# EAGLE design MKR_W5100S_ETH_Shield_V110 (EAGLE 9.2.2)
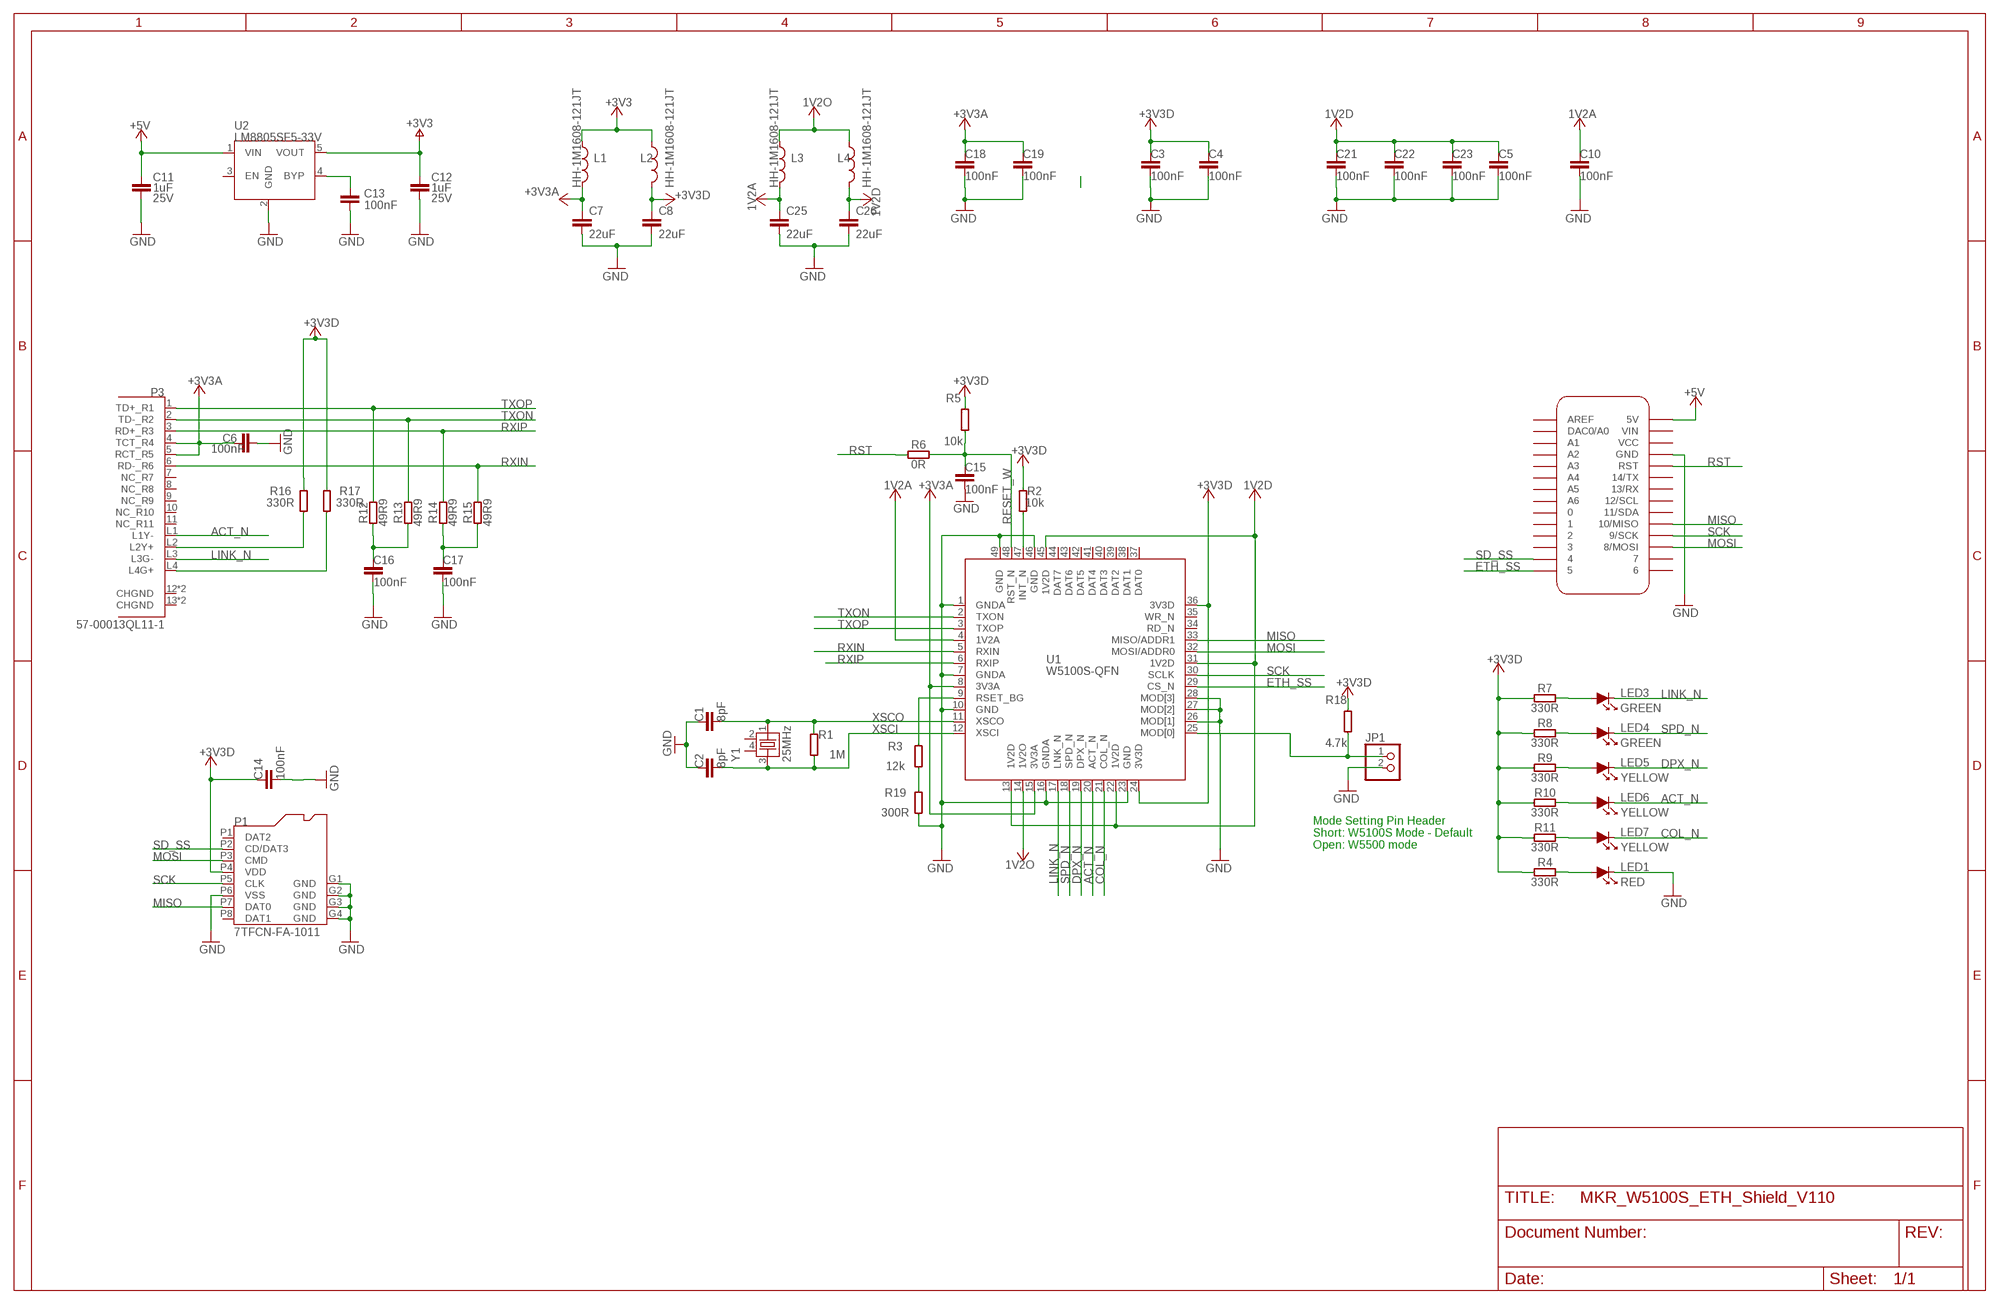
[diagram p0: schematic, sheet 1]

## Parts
C1  8pF  C-1UF-0402  [0402-1005X55N]
C2  8pF  C-1UF-0402  [0402-1005X55N]
C3  100nF  C-1UF-0402  [0402-1005X55N]
C4  100nF  C-1UF-0402  [0402-1005X55N]
C5  100nF  C-1UF-0402  [0402-1005X55N]
C6  100nF  C-1UF-0402  [0402-1005X55N]
C7  22uF  C-22U-0805  [0805-R2013X50N]
C8  22uF  C-22U-0805  [0805-R2013X50N]
C10  100nF  C-1UF-0402  [0402-1005X55N]
C11  1uF  C-1UF-0402  [0402-1005X55N]
C12  1uF  C-1UF-0402  [0402-1005X55N]
C13  100nF  C-100NF-0402  [0402-1005X55N]
C14  100nF  C-1UF-0402  [0402-1005X55N]
C15  100nF  C-1UF-0402  [0402-1005X55N]
C16  100nF  C-1UF-0402  [0402-1005X55N]
C17  100nF  C-1UF-0402  [0402-1005X55N]
C18  100nF  C-1UF-0402  [0402-1005X55N]
C19  100nF  C-1UF-0402  [0402-1005X55N]
C21  100nF  C-1UF-0402  [0402-1005X55N]
C22  100nF  C-1UF-0402  [0402-1005X55N]
C23  100nF  C-1UF-0402  [0402-1005X55N]
C25  22uF  C-22U-0805  [0805-R2013X50N]
C26  22uF  C-22U-0805  [0805-R2013X50N]
JP1  PINHD-1X2  [1X02]
L1  HH-1M1608-121JT  BLM18PG471SN1D  [0603-1608X90N]
L2  HH-1M1608-121JT  BLM18PG471SN1D  [0603-1608X90N]
L3  HH-1M1608-121JT  BLM18PG471SN1D  [0603-1608X90N]
L4  HH-1M1608-121JT  BLM18PG471SN1D  [0603-1608X90N]
LED1  RED  LED-1608  [LED-1608]
LED3  GREEN  LED-1608  [LED-1608]
LED4  GREEN  LED-1608  [LED-1608]
LED5  YELLOW  LED-1608  [LED-1608]
LED6  YELLOW  LED-1608  [LED-1608]
LED7  YELLOW  LED-1608  [LED-1608]
MKR1  DNP  ARDUINO-UTILITY_MKRBOARDNO-OUTLINE  [ARDUINO-UTILITY_MKRBOARD-NOOUTLINE]
P1  7TFCN-FA-1011  [7TFCN-FA-1011]
P3  57-00013QL11-1  [57-00013QL11-1]
R1  1M  R-330R-0402  [0402-1005X55N]
R2  10k  R-330R-0402  [0402-1005X55N]
R3  12k  R-330R-0402  [0402-1005X55N]
R4  330R  R-330R-0402  [0402-1005X55N]
R5  10k  R-330R-0402  [0402-1005X55N]
R6  0R  R-330R-0402  [0402-1005X55N]
R7  330R  R-330R-0402  [0402-1005X55N]
R8  330R  R-330R-0402  [0402-1005X55N]
R9  330R  R-330R-0402  [0402-1005X55N]
R10  330R  R-330R-0402  [0402-1005X55N]
R11  330R  R-330R-0402  [0402-1005X55N]
R12  49R9  R-330R-0402  [0402-1005X55N]
R13  49R9  R-330R-0402  [0402-1005X55N]
R14  49R9  R-330R-0402  [0402-1005X55N]
R15  49R9  R-330R-0402  [0402-1005X55N]
R16  330R  R-330R-0402  [0402-1005X55N]
R17  330R  R-330R-0402  [0402-1005X55N]
R18  4.7k  R-330R-0402  [0402-1005X55N]
R19  300R  R-330R-0402  [0402-1005X55N]
U1  W5100S-QFN  [W5100S-QFN]
U2  LM8805SF5-33V  [SOT23-5L]
Y1  25MHz  XTAL3225  [XTAL3225]

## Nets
1V2A: C10.1 C25.1 L3.2 U1.4(1V2A)
1V2D: C5.1 C21.1 C22.1 C23.1 C26.1 L4.2 U1.13(1V2D) U1.22(1V2D) U1.31(1V2D) U1.45(1V2D)
1V2O: L3.1 L4.1 U1.14(1V2O)
+3V3 [power]: C12.1 L1.1 L2.1 U2.5(VOUT)
+3V3A [power]: C6.1 C7.1 C18.1 C19.1 L1.2 P3.4(TCT_R4) P3.5(RCT_R5) U1.8(3V3A) U1.15(3V3A)
+3V3D: C3.1 C4.1 C8.1 C14.1 L2.2 P1.P4(VDD) R2.1 R4.2 R5.2 R7.2 R8.2 R9.2 R10.2 R11.2 R16.1 R17.1 R18.2 U1.24(3V3D) U1.36(3V3D)
+5V: C11.1 MKR1.5V U2.1(VIN)
ACT_N: LED6.K P3.L1(L1Y-) U1.20(ACT_N)
COL_N: LED7.K U1.21(COL_N)
DPX_N: LED5.K U1.19(DPX_N)
ETH_SS: MKR1.5 U1.29(CS_N)
GND [gnd]: C1.1 C2.1 C3.2 C4.2 C5.2 C6.2 C7.2 C8.2 C10.2 C11.2 C12.2 C13.2 C14.2 C15.2 C16.2 C17.2 C18.2 C19.2 C21.2 C22.2 C23.2 C25.2 C26.2 JP1.2 LED1.K MKR1.GND P1.G1(GND) P1.G2(GND) P1.G3(GND) P1.G4(GND) P1.P6(VSS) R19.1 U1.1(GNDA) U1.7(GNDA) U1.10(GND) U1.16(GNDA) U1.23(GND) U1.26(MOD[1]) U1.27(MOD[2]) U1.28(MOD[3]) U1.46(GND) U1.49(GND) U2.2(GND)
LINK_N: LED3.K P3.L3(L3G-) U1.17(LNK_N)
MISO: MKR1.10(10/MISO) P1.P7(DAT0) U1.33(MISO/ADDR1)
MOSI: MKR1.8(8/MOSI) P1.P3(CMD) U1.32(MOSI/ADDR0)
N$1: LED3.A R7.1
N$2: P3.L2(L2Y+) R16.2
N$3: LED1.A R4.1
N$4: LED4.A R8.1
N$5: LED5.A R9.1
N$6: LED6.A R10.1
N$7: LED7.A R11.1
N$8: P3.L4(L4G+) R17.2
N$9: JP1.1 R18.1 U1.25(MOD[0])
N$11: C13.1 U2.4(BYP)
N$12: C16.1 R12.2 R13.2
N$13: R3.1 R19.2
N$15: C17.1 R14.2 R15.2
N$16: R2.2 U1.47(INT_N)
N$20: R3.2 U1.9(RSET_BG)
RESET_W: C15.1 R5.1 R6.1 U1.48(RST_N)
RST: MKR1.RST R6.2
RXIN: P3.6(RD-_R6) R15.1 U1.5(RXIN)
RXIP: P3.3(RD+_R3) R14.1 U1.6(RXIP)
SCK: MKR1.9(9/SCK) P1.P5(CLK) U1.30(SCLK)
SD_SS: MKR1.4 P1.P2(CD/DAT3)
SPD_N: LED4.K U1.18(SPD_N)
TXON: P3.2(TD-_R2) R13.1 U1.2(TXON)
TXOP: P3.1(TD+_R1) R12.1 U1.3(TXOP)
XSCI: C2.2 R1.1 U1.12(XSCI) Y1.3
XSCO: C1.2 R1.2 U1.11(XSCO) Y1.1
Unconnected: MKR1.0 MKR1.1 MKR1.2 MKR1.3 MKR1.6 MKR1.7 MKR1.11(11/SDA) MKR1.12(12/SCL) MKR1.13(13/RX) MKR1.14(14/TX) MKR1.A0(DAC0/A0) MKR1.A1 MKR1.A2 MKR1.A3 MKR1.A4 MKR1.A5 MKR1.A6 MKR1.AREF MKR1.VCC MKR1.VIN P1.P1(DAT2) P1.P8(DAT1) P3.7(NC_R7) P3.8(NC_R8) P3.9(NC_R9) P3.10(NC_R10) P3.11(NC_R11) P3.12(CHGND) P3.13(CHGND) P3.P$3(CHGND) P3.P$4(CHGND) U1.34(RD_N) U1.35(WR_N) U1.37(DAT0) U1.38(DAT1) U1.39(DAT2) U1.40(DAT3) U1.41(DAT4) U1.42(DAT5) U1.43(DAT6) U1.44(DAT7) U2.3(EN) Y1.2 Y1.4

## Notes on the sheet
- Mode Setting Pin Header
  Short: W5100S Mode - Default
  Open: W5500 mode

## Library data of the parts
C1-C6 C10-C12 C14-C19 C21-C23 = MK1_Zero:C: Capacitor; DESCR: CAP CER 1UF 25V 10% X5R 0402; MF: Murata; MPN: GRM155R61E105KA12D; VOLTAGE: 25V
C7 C8 C25 C26 = Arduino-rcl:C: SMD Capacitor; CODE-ARDUINO: 2233; DATASHEET: https://media.digikey.com/pdf/Data%20Sheets/Samsung%20PDFs/CL21A226MQCLQNC_character.pdf; DISTRIBUTOR-LINK: https://www.digikey.com/product-detail/en/samsung-electro-mechanics-america-inc/CL21A226MQCLQNC/1276-2412-1-ND/3890498; DISTRIBUTOR-PN: 1276-2412-1-ND; MANUFACTURER: Samsung; MANUFACTURER-PN: CL21A226MQCLQNC; VALUE: 22u
C13 = MK1_Zero:C: Capacitor; DESCR: CAP CER 0.1UF 50V 10% X5R 0402; MF: TDK; MPN: C1005X5R1H104K050BB
JP1 = PinHeader:PINHD-1X2: PIN HEADER
L1-L4 = MK1_Zero:BLM18PG471SN1D: FERRITE CHIP 470 OHM 1000MA 0603
LED1 LED3-LED7 = DIODE:LED-1608
MKR1 = MKRETHShieldV2.0:ARDUINO-UTILITY_MKRBOARD: MKR board footprint; DATASHEET: DNP; DISTRIBUTOR-LINK: DNP; DISTRIBUTOR-PN: DNP; MANUFACTURER: DNP; MANUFACTURER-PN: DNP
P1 = Connector:7TFCN-FA-1011
P3 = WIZnet:57-00013QL11-1
R1-R19 = MK1_Zero:R: Resistor; DESCR: RES 330 OHM 1/16W 1% 0402 SMD; MF: Yageo; MPN: RC0402FR-07330RL
U1 = WIZnet:W5100S-QFN
U2 = RECULATOR:LM8805SF5-33V
Y1 = X-TAL:XTAL3225

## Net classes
1 power: width 0.254 mm, drill 0.3 mm, clearance 0.127 mm
2 gnd: width 0.254 mm, drill 0.3 mm, clearance 0.127 mm

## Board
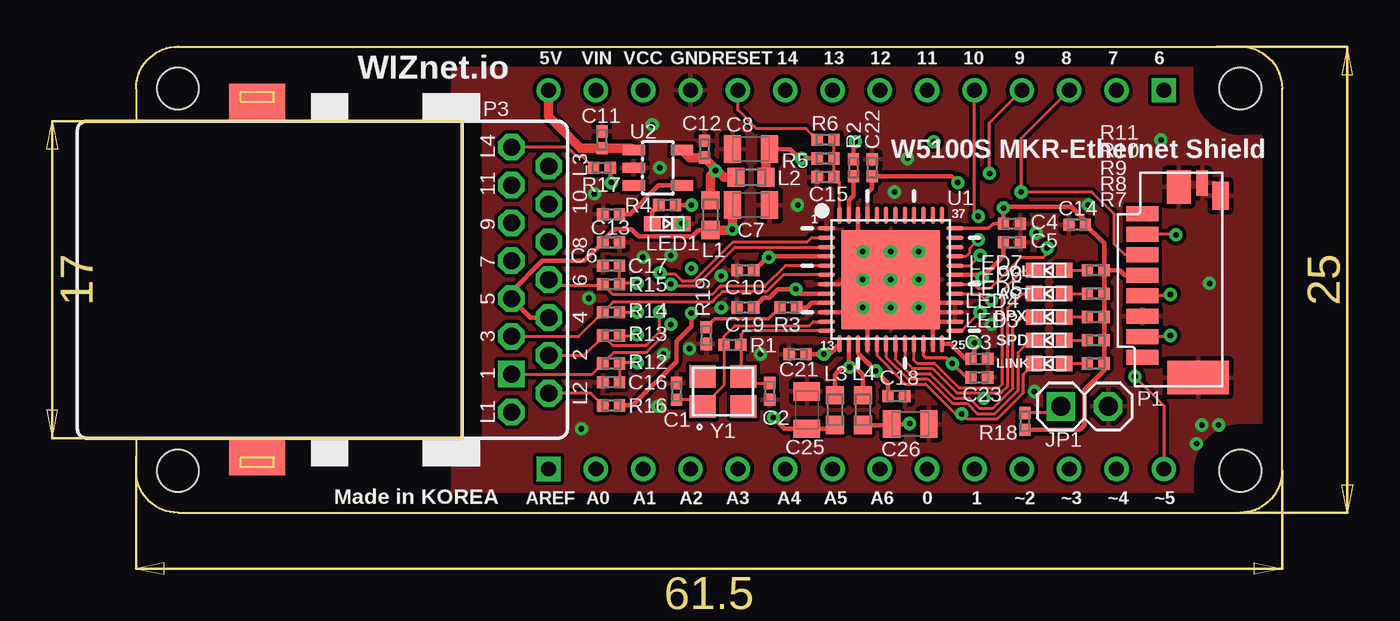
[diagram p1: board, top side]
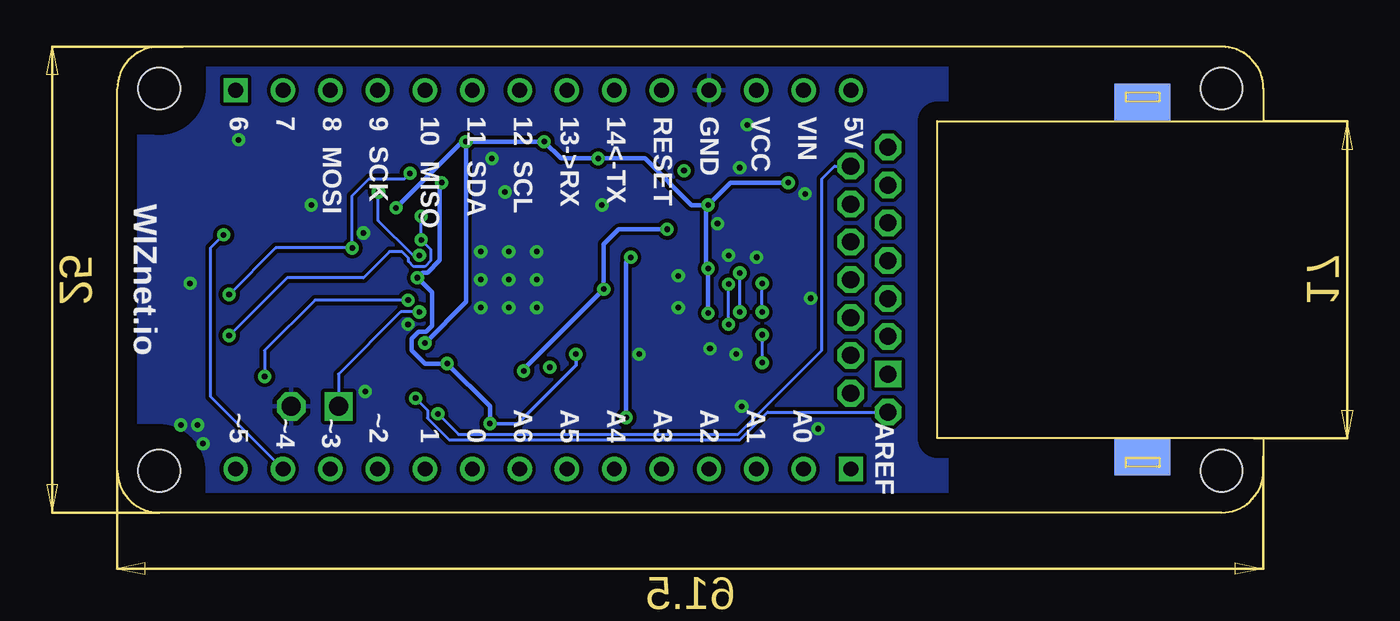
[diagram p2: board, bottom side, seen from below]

Size 70.1 x 28.3 mm. Coordinates in mm from the lower left corner, seen from the top.
Outline: 7.05,3.3 64.05,3.3 arc90 66.3,5.55 66.3,26.05 arc90 64.05,28.3 7.05,28.3 arc90 4.8,26.05 4.8,24.3 22.3,24.3 22.3,7.3 4.8,7.3 4.8,5.55 arc90 7.05,3.3
Copper layers (1*16): Top 0.035mm / dielectric 1.5mm / Bottom 0.035mm
Design rules "default *": minimum track width 6mil, minimum drill 0.3mm, track to track 5mil, track to pad 5mil, pad to pad 5mil, via to via 5mil, smd to smd 5mil, copper to edge 40mil, drill to drill 6mil, minimum pad ring 10mil, minimum via ring 8mil, stop-mask expansion 4mil, vias tented up to drill 15mil, thermal gap 10mil
Holes 2.25 mm at 7.05,5.55 7.05,26.05 64.05,5.55 64.05,26.05
tRestrict: area 61.8,23.8 to 66.3,28.3; area 61.8,3.3 to 66.3,7.8; 4 lines
bRestrict: area 61.8,23.8 to 66.3,28.3; area 61.8,3.3 to 66.3,7.8; 4 lines

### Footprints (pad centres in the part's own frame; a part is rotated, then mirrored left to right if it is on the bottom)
0402-1005X55N = smd 0.62 x 0.62: 1 -0.45,0; 2 0.45,0
0805-R2013X50N = smd 0.95 x 1.45: 1 -1,0; 2 1,0
1X02 = drill 1.016 square: 1 -1.27,0 | drill 1.016 octagon: 2 1.27,0
0603-1608X90N = smd 0.95 x 1: 1 -0.8,0; 2 0.8,0
LED-1608 = smd 0.89 x 0.82: A -0.8,0; K 0.8,0
ARDUINO-UTILITY_MKRBOARD-NOOUTLINE = drill 0.8: 0 42.455,2.34; 1 44.995,2.34; 2 47.535,2.34; 3 50.075,2.34; 4 52.615,2.34; 5 55.155,2.34; 5V 22.135,22.66; 7 52.615,22.66; 8 50.075,22.66; 9 47.535,22.66; 10 44.995,22.66; 11 42.455,22.66; 12 39.915,22.66; 13 37.375,22.66; 14 34.835,22.66; A0 24.675,2.34; A1 27.215,2.34; A2 29.755,2.34; A3 32.295,2.34; A4 34.835,2.34; A5 37.375,2.34; A6 39.915,2.34; GND 29.755,22.66; RST 32.295,22.66; VCC 27.215,22.66; VIN 24.675,22.66 | drill 0.8 square: 6 55.155,22.66; AREF 22.135,2.34
7TFCN-FA-1011 = smd 1.8 x 3.3: G1 -5.26,0 | smd 1.8 x 1.3: G2 4.97,1.04 | smd 1.36 x 0.6: G3 5.19,-0.21 | smd 1.5 x 0.9: G4 4.49,-1.2 | smd 0.8 x 1.7: P1 3.54,3; P2 2.44,3; P3 1.34,3; P4 0.24,3; P5 -0.86,3; P6 -1.96,3; P7 -3.06,3; P8 -4.16,3
57-00013QL11-1 = drill 0.914 square: 1 5.075,10.15 | drill 0.914 octagon: 2 4.065,12.15; 3 3.045,10.15; 4 2.035,12.15; 5 1.015,10.15; 6 0.005,12.15; 7 -1.015,10.15; 8 -2.025,12.15; 9 -3.045,10.15; 10 -4.055,12.15; 11 -5.075,10.15; L1 7.105,10.15; L2 6.095,12.15; L3 -6.085,12.15; L4 -7.105,10.15 | smd 2 x 3: 12 -9.5,-3.51; 13 9.5,-3.51 | smd 2 x 3 bottom: P$3 -9.5,-3.51; P$4 9.5,-3.51
W5100S-QFN = smd 0.95 x 0.25: 1 -3.45,2.75; 2 -3.45,2.25; 3 -3.45,1.75; 4 -3.45,1.25; 5 -3.45,0.75; 6 -3.45,0.25; 7 -3.45,-0.25; 8 -3.45,-0.75; 9 -3.45,-1.25; 10 -3.45,-1.75; 11 -3.45,-2.25; 12 -3.45,-2.75; 25 3.45,-2.75; 26 3.45,-2.25; 27 3.45,-1.75; 28 3.45,-1.25; 29 3.45,-0.75; 30 3.45,-0.25; 31 3.45,0.25; 32 3.45,0.75; 33 3.45,1.25; 34 3.45,1.75; 35 3.45,2.25; 36 3.45,2.75 | smd 0.25 x 0.95: 13 -2.75,-3.45; 14 -2.25,-3.45; 15 -1.75,-3.45; 16 -1.25,-3.45; 17 -0.75,-3.45; 18 -0.25,-3.45; 19 0.25,-3.45; 20 0.75,-3.45; 21 1.25,-3.45; 22 1.75,-3.45; 23 2.25,-3.45; 24 2.75,-3.45; 37 2.75,3.45; 38 2.25,3.45; 39 1.75,3.45; 40 1.25,3.45; 41 0.75,3.45; 42 0.25,3.45; 43 -0.25,3.45; 44 -0.75,3.45; 45 -1.25,3.45; 46 -1.75,3.45; 47 -2.25,3.45; 48 -2.75,3.45 | smd 5.3 x 5.3: 49 0,0
SOT23-5L = smd 0.55 x 1.2: 1 -0.95,-1.3; 2 0,-1.3; 3 0.95,-1.3; 4 0.95,1.3; 5 -0.95,1.3
XTAL3225 = smd 1.4 x 1.2: 1 -1.1,-0.8; 2 1.1,-0.8; 3 1.1,0.8; 4 -1.1,0.8

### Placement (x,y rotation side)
C1  33.8,9.8 270 top
C2  38.8,9.8 90 top
C3  50.05,11.55 0 top
C4  51.8,18.8 0 top
C5  51.8,17.8 0 top
C6  30.3,17.8 0 top
C7  37.8,19.8 0 top
C8  37.8,22.8 180 top
C10  37.5,16.3 180 top
C11  29.8,23.3 90 top
C12  35.3,22.8 90 top
C13  30.3,19.3 180 top
C14  55.3,18.75 180 top
C15  41.8,21.3 180 top
C16  30.3,10.3 180 top
C17  30.3,16.55 180 top
C18  45.6,9.55 0 top
C19  37.5,14.3 180 top
C21  40.3,11.8 180 top
C22  44.3,21.8 90 top
C23  50.05,10.55 0 top
C25  40.8,8.8 90 top
C26  46.35,8.05 0 top
JP1  55.7,9 0 top
L1  35.63,19.26 270 top
L2  37.8,21.3 0 top
L3  42.3,8.8 270 top
L4  43.8,8.8 270 top
LED1  33.3,18.8 0 top
LED3  53.8,11.3 180 top
LED4  53.8,12.55 180 top
LED5  53.8,13.8 180 top
LED6  53.8,15.05 180 top
LED7  53.8,16.3 180 top
MKR1  4.8,3.3 0 top
P1  61.8,15.8 90 top
P3  14.8,15.8 270 top
R1  36.8,12.3 180 top
R2  43.3,21.8 270 top
R3  39.8,14.3 0 top
R4  33.3,19.8 0 top
R5  41.8,22.3 180 top
R6  41.8,23.3 180 top
R7  56.3,11.3 0 top
R8  56.3,12.55 0 top
R9  56.3,13.8 0 top
R10  56.3,15.05 0 top
R11  56.3,16.3 0 top
R12  30.3,11.3 0 top
R13  30.3,12.8 0 top
R14  30.3,14.05 0 top
R15  30.3,15.55 0 top
R16  30.3,9.05 180 top
R17  29.8,21.8 180 top
R18  52.5,8.2 270 top
R19  35.4,12.8 90 top
U1  45.3,15.8 0 top
U2  32.8,21.8 270 top
Y1  36.3,9.8 0 top

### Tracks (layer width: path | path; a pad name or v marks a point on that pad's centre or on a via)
1V2A  (via drill 0.3)
  Top 0.152: v38.75,16.99 38.75,17.05
  Top 0.254: U1.4 38.75,17.05 38,16.3 C10.1 | L3.2 42.1,7.8 C25.1 39.6,7.8 v39,8.4
  Bottom 0.254: v39,8.4 39,16.74 v38.75,16.99
1V2D  (via drill 0.3)
  Top 0.2: U1.22 47.05,11.75 47.18,11.62 48.28,11.62 v48.6,11.3 49.35,10.55 49.5,10.55 | 46.28,8.05 v46.31,8.08
  Top 0.254: U1.13 42,11.8 v41.7,11.8 C21.1 | 49.5,10.55 C23.1 | L4.2 45.3,8 C26.1 46.28,8.05 | U1.45 44.05,20.45 44.3,20.7 C22.1 48.55,21.35 v48.9,21 | U1.31 50.05,16.05 v50.2,15.9 51.35,17.05 C5.1
  Bottom 0.2: v46.31,8.08 44.82,8.08 41.7,11.2 v41.7,11.8
  Bottom 0.25: 50.5,12.64 50.14,13 49.73,13 49.42,13.32 49.42,15.12 49.79,15.49
  Bottom 0.254: v46.31,8.08 46.31,9.01 v48.6,11.3 49.8,11.3 50.5,12 50.5,12.64 | v48.9,21 49,20.9 49,16.83 49.66,16.17 49.93,16.17 v50.2,15.9 49.79,15.49
1V2O  (via drill 0.3)
  Top 0.254: U1.14 43.05,11.15 v43.1,11.1 | v43.1,11.1 42.7,11.1 42.3,10.7 L3.1 | v43.1,11.1 43.4,11.1 43.8,10.7 L4.1
+3V3  (via drill 0.3)
  Top 0.508: U2.5 34.5,22.35 C12.1 36.02,21.62 | 36.02,21.62 36.35,21.3 L2.1 | 36.02,21.62 | 36.02,21.62 35.91,21.62 v35.89,21.64 35.63,21.38 L1.1
+3V3A  (via drill 0.3)
  Top 0.254: U1.15 43.55,11.85 v44.5,10.9 45.15,10.25 C18.1 | U1.8 40.44,15.05 v40.2,15.29 39.24,15.29 38.78,14.83 38.48,14.83 C19.1 | L1.2 34.97,18.46 34.65,18.14 31.76,18.14 31.4,18.5 30.48,18.5 29.85,17.87 C6.1 28.85,16.8 26.59,16.8 24.95,15.16 P3.5 25.97,13.77 P3.4
  Top 0.508: L1.2 36.76,18.46 | 36.76,18.46 v36.8,18.5 | C7.1 v36.8,18.5 | v36.8,18.5 36.76,18.46
  Bottom 0.254: v36.8,18.5 39.4,18.5 40.2,17.7 v40.2,15.29 44.5,10.99 v44.5,10.9
+3V3D  (via drill 0.3)
  Top 0.152: v51.35,19.65 51.35,19.7
  Top 0.2: U1.36 50.55,18.55 50.8,18.8 C4.1
  Top 0.254: U1.24 48.5,12.35 49.3,11.55 C3.1 49.6,11.7 49.8,11.9 v49.8,12.4 | R11.2 R10.2 R9.2 R8.2 R7.2 56.75,10.95 55.7,9.9 55.7,8 55.45,7.75 R18.2 | P1.P4 57.86,16.04 57.6,16.3 R11.2 | R11.2 56.75,17.75 C14.1 55.75,18.95 55,19.7 51.35,19.7 C4.1 | R17.1 30.25,21.05 v30.3,21 | v34.6,19.8 R4.2 | C8.1 39.9,22.8 40.4,22.3 v40.5,22.3 R5.2 | v43.4,23.2 43.3,23.1 R2.1 | 34.6,14.1 v34.6,14 34.6,13.3 33.8,12.5 33.8,11.4 31.45,9.05 R16.1
  Top 0.508: L2.2 38.6,22.6 C8.1
  Bottom 0.254: v30.3,21 33.4,21 v34.6,19.8 34.71,19.8 | 34.71,19.8 35.5,19.8 38,22.3 v40.5,22.3 42.5,22.3 v43.4,23.2 v47.6,23.2 | v47.6,23.2 47.8,23.2 v51.35,19.65 | v49.8,12.4 47.6,14.6 v47.6,23.2 | v34.6,14 v34.6,16.4 34.71,16.51 34.71,19.8
+5V
  Top 0.508: U2.1 31.4,22.85 C11.1 28.65,22.85 26.94,24.57 MKR1.5V
ACT_N  (via drill 0.3)
  Top 0.152: 46.05,11.99 U1.20 46.05,11.45 46.46,11.04 47.52,11.04 48.84,9.72 50.02,9.72 v50.3,9.44 50.58,9.72 51.22,9.72 51.58,10.08 51.58,14.28 52.35,15.05 LED6.K
  Bottom 0.152: v50.3,9.44 49.66,8.8 49.66,8.37 48.51,7.22 32.88,7.22 31.41,8.7 P3.L1
COL_N
  Top 0.152: U1.21 46.55,11.47 46.7,11.32 47.64,11.32 48.58,10.37 | 48.58,10.37 48.68,10.28 | 48.68,10.28 48.73,10.23 48.58,10.37 | 48.68,10.28 48.96,10 51.1,10 51.3,10.2 51.3,15.2 52.4,16.3 LED7.K
DPX_N
  Top 0.152: 45.55,11.98 U1.19 45.55,11.54 46.33,10.76 47.41,10.76 48.72,9.44 49.52,9.44 50.07,8.89 50.78,8.89 51.86,9.97 51.86,13.26 52.4,13.8 LED5.K
ETH_SS  (via drill 0.3)
  Top 0.152: U1.29 50.05,15.05 50.4,14.7 v50.7,14.7 | v58.4,10.6 59.95,9.04 MKR1.5
  Bottom 0.152: v50.7,14.7 55.7,14.7 58.4,12 v58.4,10.6
GND  (via drill 0.3)
  Top 0.254: U1.28 47.05,14.55 46.9,14.4 | 46.9,14.4 v46.8,14.3 | U1.46 43.55,17.55 v43.8,17.3 | U1.10 43.55,14.05 v43.8,14.3 44.05,14.05 U1.16 | U1.7 43.55,15.55 v43.8,15.8 | U1.23 47.55,13.64 | 47.55,13.64 47.55,13.75 47.45,13.85 | 47.45,13.85 46.9,14.4 | U1.27 47.65,14.05 47.45,13.85 | U1.26 47.64,13.55 47.55,13.64
  other vias: 45.3,15.8 45.3,14.3 45.3,17.3 46.8,15.8 46.8,17.3 53.1,18.3 55.9,19.8 40.3,19.8 45.5,20.5 38.3,11.8 32,17 32.9,21.8 34.1,18.8 29.4,20.4 29.1,14.8 33.1,11.8 36.2,16 62,8 62.9,8 61.7,7 62.4,15.6 59.8,23.3 32.5,24.1 28.7,7.8 32.8,9 33.5,17.1 46.2,22.3 53,9.8 50.7,13.4 36.2,14.3 34.5,12.1
  pour Top (isolate 0.2): 21.8,2.3 21.8,29.3 66.8,29.3 66.8,2.3
  pour Bottom (isolate 0.2): 21.8,30.3 21.8,1.3 67.8,1.3 67.8,30.3
LINK_N  (via drill 0.3)
  Top 0.152: U1.17 44.55,11.75 46.1,10.2 47.18,10.2 48.78,8.6 v49.1,8.6 49.37,8.33 51.01,8.33 52.42,9.74 52.42,10.72 LED3.K
  Bottom 0.152: v49.1,8.6 48,7.5 33,7.5 28.5,12 28.5,21.2 27.82,21.89 P3.L3
MISO  (via drill 0.3)
  Top 0.152: v50,19.2 49.79,19.41 MKR1.10 | v60.3,12.8 60.24,12.74 P1.P7 | U1.33 49.35,17.05 49.54,17.24 49.54,17.48 v50,17.93
  Bottom 0.152: v60.3,12.8 57.2,15.9 53.1,15.9 51.7,17.3 51.03,17.3 50.68,16.95 50.68,16.78 50.4,16.5 49.8,16.5 49.5,16.8 49.5,17.43 v50,17.93 v50,19.2
MOSI  (via drill 0.3)
  Top 0.152: U1.32 49.55,16.55 v50.1,17.1 | MKR1.8 52.3,23.39 v52.3,20.5 56.1,20.5 57.3,19.3 57.3,17.7 57.86,17.14 P1.P3
  Bottom 0.152: v52.3,20.5 52.3,18.97 50.43,17.1 v50.1,17.1
N$1
  Top 0.152: R7.1 LED3.A
N$2
  Top 0.152: R16.2 29.2,9.71 P3.L2
N$3
  Top 0.254: R4.1 32.5,19.45 LED1.A
N$4
  Top 0.152: LED4.A R8.1
N$5
  Top 0.152: LED5.A R9.1
N$6
  Top 0.152: LED6.A R10.1
N$7
  Top 0.152: LED7.A R11.1
N$8
  Top 0.152: R17.2 28.76,22.39 28.46,22.39 27.95,22.91 P3.L4
N$9  (via drill 0.3)
  Top 0.152: JP1.1 54.08,8.65 R18.1 | 49.88,13.85 v50.1,14.07 49.08,13.05 U1.25
  Bottom 0.152: v50.1,14.07 51.1,14.07 54.43,10.74 JP1.1
N$11
  Top 0.254: U2.4 32.85,20.85 31.3,19.3 C13.1
N$12  (via drill 0.3)
  Top 0.152: R13.2 31.66,12.8 v31.7,12.84 | v31.7,11.34 30.79,11.34 R12.2 C16.1
  Bottom 0.152: v31.7,12.84 v31.7,11.34
N$13
  Top 0.2: R3.1 38.75,13.7 35.85,13.7 R19.2
N$15  (via drill 0.3)
  Top 0.152: R14.2 31.69,14.05 v31.7,14.06 | v31.7,15.6 30.8,15.6 R15.2 C17.1
  Bottom 0.152: v31.7,14.06 v31.7,15.6
N$16
  Top 0.254: U1.47 43.05,20.05 43.3,20.3 R2.2
N$20
  Top 0.254: U1.9 41.05,14.55 40.8,14.3 R3.2
RESET_W
  Top 0.152: U1.48 42.55,21 C15.1 R5.1 R6.1
RST
  Top 0.152: R6.2 40.75,23.9 38.1,23.9 37.09,24.91 MKR1.RST
RXIN
  Top 0.152: U1.5 39.64,16.55 38.53,15.44 36.2,15.44 | 36.2,15.44 36.14,15.44 | 36.14,15.44 | 36.2,15.44 36.14,15.44 | 36.14,15.44 35.7,15 30.4,15 30.24,15.16 29.9,15.5 | 29.9,15.5 R15.1 | P3.6 27.25,15.5 29.9,15.5
RXIP
  Top 0.152: U1.6 39.53,16.05 38.64,15.16 36.26,15.16 35.85,14.75 35.72,14.62 30.42,14.62 30.24,14.44 R14.1 28.55,12.75 P3.3
SCK  (via drill 0.3)
  Top 0.152: v60.3,15 60.24,14.94 P1.P5 | v50.6,21.5 50.6,24.23 MKR1.9 | v53.7,17.5 53.7,17.2 53.5,17 52.3,17 50.64,15.34 49.97,15.34 49.76,15.55 U1.30
  Bottom 0.152: v60.3,15 57.8,17.5 v53.7,17.5 53.7,20.3 52.8,21.2 50.9,21.2 v50.6,21.5
SD_SS  (via drill 0.3)
  Top 0.152: v60.6,18.2 60.56,18.24 P1.P2
  Bottom 0.152: MKR1.4 61.3,9.52 61.3,17.5 v60.6,18.2
SPD_N
  Top 0.152: 45.05,12 U1.18 45.05,11.64 46.22,10.48 47.29,10.48 48.61,9.16 49.4,9.16 49.95,8.61 50.89,8.61 52.14,9.85 52.14,11.9 52.79,12.55 LED4.K
TXON  (via drill 0.3)
  Top 0.152: R13.1 29.88,12.77 | 29.88,12.77 30.24,12.41 30.36,12.29 32.19,12.29 32.9,13 v32.9,14.06 | v32.9,16.16 32.94,16.11 33.73,16.11 34.1,15.75 34.75,15.75 36.83,17.83 40.83,17.83 41.05,18.05 U1.2 | P3.2 28.84,11.73 29.88,12.77
  Bottom 0.152: v32.9,14.06 v32.9,16.16
TXOP  (via drill 0.3)
  Top 0.152: U1.3 36.95,17.55 34.87,15.47 33.59,15.47 v33.5,15.56 | v33.5,13.4 33.18,13.08 33.18,12.88 32.2,11.9 30.45,11.9 30.24,11.69 R12.1 29.28,10.72 P3.1
  Bottom 0.152: v33.5,13.4 v33.5,15.56
XSCI
  Top 0.152: U1.12 37.45,13.05 37.25,12.85 R1.1 37.25,10.75 Y1.3 37.75,10.25 C2.2
XSCO
  Top 0.152: C1.2 34.85,9.35 Y1.1 35.22,9 36.35,10.13 R1.2 36.35,12.75 36.93,13.33 40.93,13.33 41.15,13.55 U1.11

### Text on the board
tNames: Y1
tsilk: 5V | VIN | VCC | GND | RESET | 14 | 13 | 12 | 11 | 10 | 9 | 8 | 7 | 6 | WIZnet.io | W5100S MKR-Ethernet Shield | COL | ACT | DPX | SPD | LINK | Made in KOREA | AREF | A0 | A1 | A2 | A3 | A4 | A5 | A6 | 0 | 1 | ~2 | ~3 | ~4 | ~5
bsilk: 5V | VIN | VCC | GND | RESET | 14<-TX | 13->RX | 12 SCL | 11 SDA | 10 MISO | 9 SCK | 8 MOSI | 7 | 6 | WIZnet.io | A0 | A1 | A2 | A3 | A4 | A5 | A6 | 0 | 1 | ~2 | ~5 | ~3 | ~4 | AREF

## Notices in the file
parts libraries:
Arduino-rcl: Copyright (c) 2016-2017 Arduino LLC. All right reserved.
